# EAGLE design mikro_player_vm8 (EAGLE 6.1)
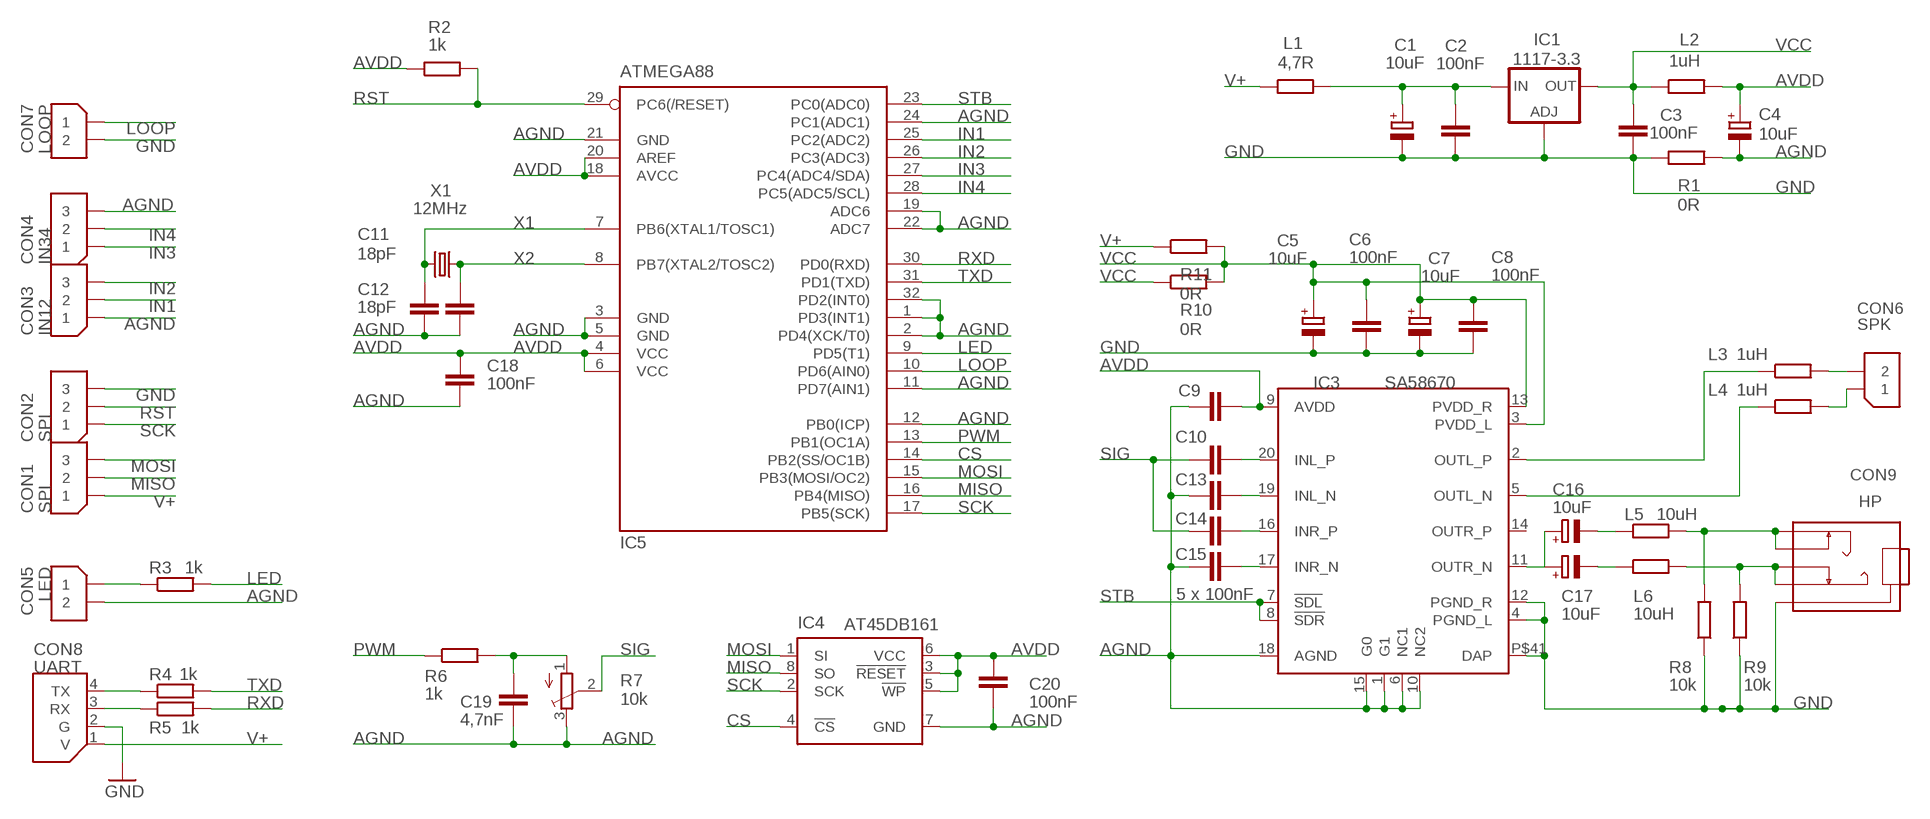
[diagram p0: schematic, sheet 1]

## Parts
C1  10uF  CPOL-EUSMCA  [SMC_A]
C2  100nF  C-EUC0805K  [C0805K]
C3  100nF  C-EUC0805K  [C0805K]
C4  10uF  CPOL-EUSMCA  [SMC_A]
C5  10uF  CPOL-EUSMCA  [SMC_A]
C6  100nF  C-EUC0805K  [C0805K]
C7  10uF  CPOL-EUSMCA  [SMC_A]
C8  100nF  C-EUC0805K  [C0805K]
C9  100nF  C-EUC0805K  [C0805K]
C10  100nF  C-EUC0805K  [C0805K]
C11  18pF  C-EUC0805K  [C0805K]
C12  18pF  C-EUC0805K  [C0805K]
C13  100nF  C-EUC0805K  [C0805K]
C14  100nF  C-EUC0805K  [C0805K]
C15  100nF  C-EUC0805K  [C0805K]
C16  10uF  CPOL-EUSMCA  [SMC_A]
C17  10uF  CPOL-EUSMCA  [SMC_A]
C18  100nF  C-EUC0805K  [C0805K]
C19  4,7nF  C-EUC0805K  [C0805K]
C20  100nF  C-EUC0805K  [C0805K]
CON1  SPI  GOLDPIN_1X3  [GOLDPIN_1X3]
CON2  SPI  GOLDPIN_1X3  [GOLDPIN_1X3]
CON3  IN12  GOLDPIN_1X3  [GOLDPIN_1X3]
CON4  IN34  GOLDPIN_1X3  [GOLDPIN_1X3]
CON5  LED  GOLDPIN_1X2  [GOLDPIN_1X2]
CON6  SPK  GOLDPIN_1X2  [GOLDPIN_1X2]
CON7  LOOP  GOLDPIN_1X2  [GOLDPIN_1X2]
CON8  UART  MOD09  [MOD09]
CON9  HP  JACK_3_5  [JACK_3_5]
IC1  1117-3.3  LD117ADT33TR  [DPACK]
IC3  SA58670  [MLF20]
IC4  AT45DB161  AT45DBXXX  [SOIC8]
IC5  ATMEGA88  MEGA8-AI  [TQFP32-08]
L1  4,7R  R-EU_R0805  [R0805]
L2  1uH  R-EU_R0805  [R0805]
L3  1uH  R-EU_R0805  [R0805]
L4  1uH  R-EU_R0805  [R0805]
L5  10uH  R-EU_R0805  [R0805]
L6  10uH  R-EU_R0805  [R0805]
R1  0R  R-EU_R0805  [R0805]
R2  1k  R-EU_R0805  [R0805]
R3  1k  R-EU_R0805  [R0805]
R4  1k  R-EU_R0805  [R0805]
R5  1k  R-EU_R0805  [R0805]
R6  1k  R-EU_R0805  [R0805]
R7  10k  TRIM_EU-SM-42/43A  [SM-42/43A]
R8  10k  R-EU_R0805  [R0805]
R9  10k  R-EU_R0805  [R0805]
R10  0R  R-EU_R0805  [R0805]
R11  0R  R-EU_R0805  [R0805]
X1  12MHz  CRYSTALHC49UP  [HC49UP]

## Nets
AGND: C4.- C9.2 C11.1 C12.1 C13.1 C15.1 C18.2 C19.2 C20.1 CON3.P$1 CON4.P$3 CON5.2 IC3.1(G1) IC3.6(NC1) IC3.10(NC2) IC3.15(G0) IC3.18(AGND) IC4.7(GND) IC5.1(PD3(INT1)) IC5.2(PD4(XCK/T0)) IC5.3(GND) IC5.5(GND) IC5.11(PD7(AIN1)) IC5.12(PB0(ICP)) IC5.19(ADC6) IC5.21(GND) IC5.22(ADC7) IC5.24(PC1(ADC1)) IC5.32(PD2(INT0)) R1.2 R7.3(E)
AVDD: C4.+ C9.1 C18.1 C20.2 IC3.9(AVDD) IC4.3(!RESET) IC4.5(!WP) IC4.6(VCC) IC5.4(VCC) IC5.6(VCC) IC5.18(AVCC) IC5.20(AREF) L2.2 R2.1
CS: IC4.4(!CS) IC5.14(PB2(SS/OC1B))
GND: C1.- C2.2 C3.2 C5.- C6.2 C7.- C8.2 CON2.P$3 CON7.2 CON8.2(G) CON9.G IC1.1(ADJ) IC3.4(PGND_L) IC3.12(PGND_R) IC3.P$41(DAP) R1.1 R8.1 R9.1
IN1: CON3.P$2 IC5.25(PC2(ADC2))
IN2: CON3.P$3 IC5.26(PC3(ADC3))
IN3: CON4.P$1 IC5.27(PC4(ADC4/SDA))
IN4: CON4.P$2 IC5.28(PC5(ADC5/SCL))
LED: IC5.9(PD5(T1)) R3.2
LOOP: CON7.1 IC5.10(PD6(AIN0))
MISO: CON1.P$2 IC4.8(SO) IC5.16(PB4(MISO))
MOSI: CON1.P$3 IC4.1(SI) IC5.15(PB3(MOSI/OC2))
N$1: CON8.4(TX) R4.1
N$2: CON8.3(RX) R5.1
N$5: C10.2 IC3.20(INL_P)
N$6: CON5.1 R3.1
N$7: C13.2 IC3.19(INL_N)
N$8: C14.2 IC3.16(INR_P)
N$9: C15.2 IC3.17(INR_N)
N$12: C17.- L6.1
N$13: C16.- L5.1
N$14: CON6.2 L3.2
N$15: CON6.1 L4.2
N$16: CON9.R CON9.RW L5.2 R8.2
N$17: IC3.2(OUTL_P) L3.1
N$18: IC3.5(OUTL_N) L4.1
N$19: C19.1 R6.2 R7.1(A)
N$22: CON9.L CON9.LW L6.2 R9.2
N$32: C16.+ C17.+ IC3.11(OUTR_N)
PVCC: C1.+ C2.1 IC1.3(IN) L1.2
PWM: IC5.13(PB1(OC1A)) R6.1
RST: CON2.P$2 IC5.29(PC6(/RESET)) R2.2
RXD: IC5.30(PD0(RXD)) R5.2
SCK: CON2.P$1 IC4.2(SCK) IC5.17(PB5(SCK))
SIG: C10.1 C14.1 R7.2(S)
STB: IC3.7(!SDL) IC3.8(!SDR) IC5.23(PC0(ADC0))
TXD: IC5.31(PD1(TXD)) R4.2
V+: CON1.P$1 CON8.1(V) L1.1 R11.1
VCC: C3.1 C5.+ C6.1 C7.+ C8.1 IC1.4(OUT) IC3.3(PVDD_L) IC3.13(PVDD_R) L2.1 R10.1 R10.2 R11.2
X1: C11.2 IC5.7(PB6(XTAL1/TOSC1)) X1.2
X2: C12.2 IC5.8(PB7(XTAL2/TOSC2)) X1.1
Unconnected: IC3.14(OUTR_P)

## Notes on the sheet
- 5 x 100nF

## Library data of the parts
C1 C4 C5 C7 C16 C17 = rcl:CPOL-EU: POLARIZED CAPACITOR, European symbol
C2 C3 C6 C8-C15 C18-C20 = rcl:C-EU: CAPACITOR, European symbol
CON1-CON4 = DS:GOLDPIN_1X3
CON5-CON7 = DS:GOLDPIN_1X2
CON8 = DS:MOD09
CON9 = Jacki:JACK_3_5
IC1 = v-reg:LD117A?*: Low drop fixed and adjustable positive voltage regulators 1 A Source: http://www.st.com/stonline/products/literature/ds/7194/ld1117axx.pdf
IC3 = DS:SA58670
IC4 = DS:AT45DBXXX
IC5 = atmel:MEGA8: MICROCONTROLLER 8 Kbytes FLASH, 1 kbytes SRAM, 512 bytes EEPROM, USART, 6-channel 10 bit ADC, 2-channel 8 bit ADC Pin compatible with Atmega48, ATMega88, ATMega168 Source: avr.lbr; MPN: ATMEGA8-16AU; OC_FARNELL: 9171371; OC_NEWARK: 73M8863
L1-L6 R1-R6 R8-R11 = rcl:R-EU_: RESISTOR, European symbol
R7 = pot:TRIM_EU-: POTENTIOMETER
X1 = crystal:CRYSTAL: CRYSTAL; OC_FARNELL: unknown; OC_NEWARK: unknown

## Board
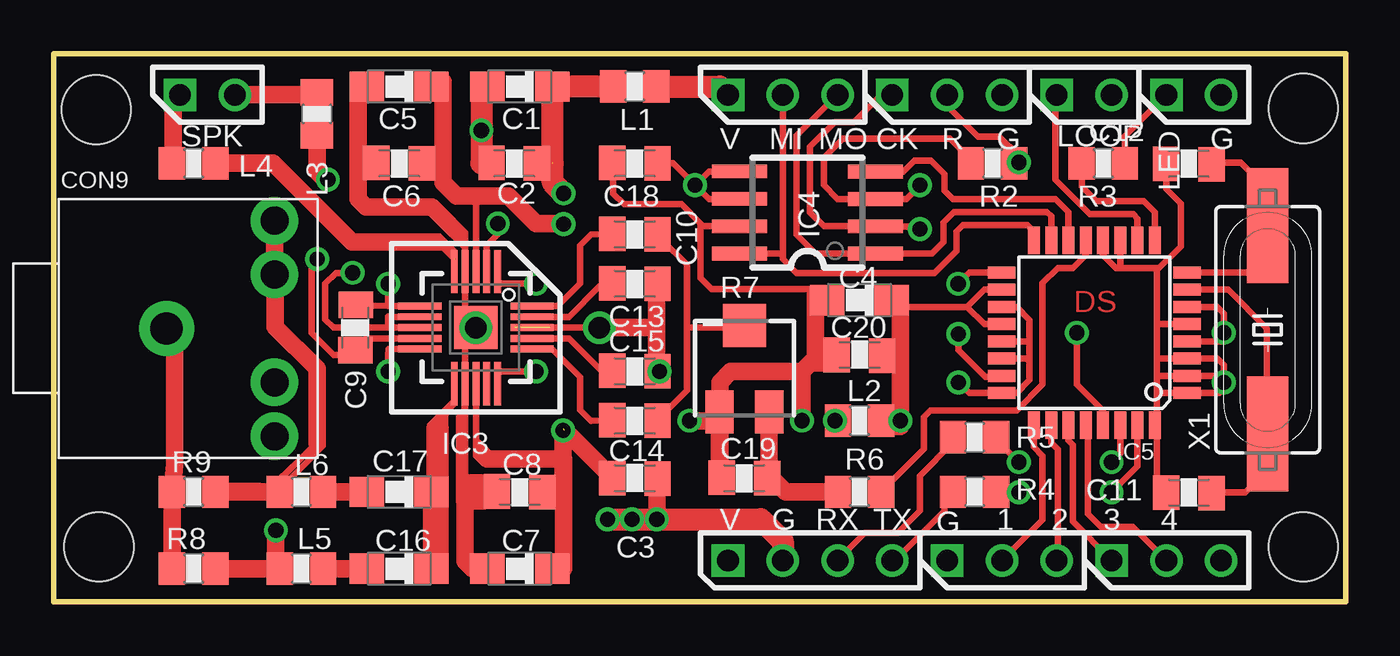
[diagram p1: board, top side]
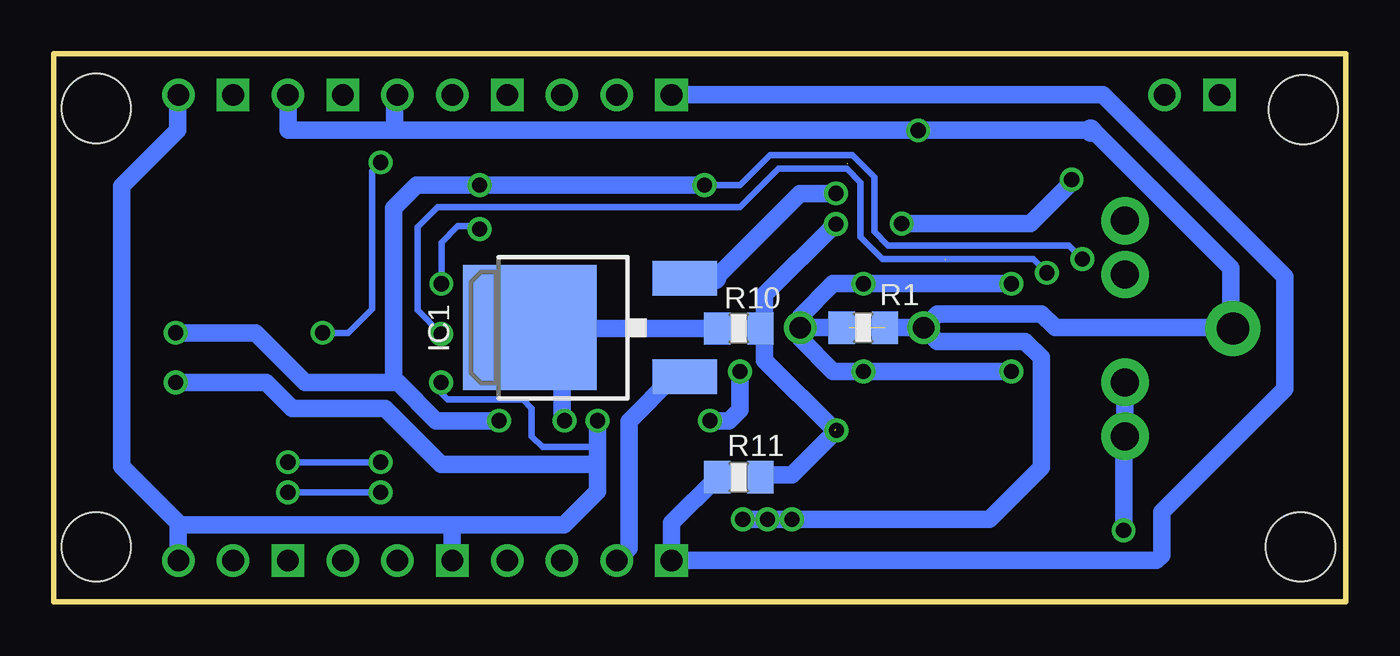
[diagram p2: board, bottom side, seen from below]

Size 59.87 x 25.42 mm. Coordinates in mm from the lower left corner, seen from the top.
Outline: 0,0 59.87,0 59.87,25.42 0,25.42 0,0
Copper layers (1*16): Top 0.035mm / dielectric 1.5mm / Bottom 0.035mm
Design rules: minimum track width 10mil, minimum drill 24mil, track to track 8mil, track to pad 8mil, pad to pad 8mil, via to via 8mil, smd to smd 8mil, copper to edge 40mil, drill to drill 8mil, minimum pad ring 10mil, minimum via ring 8mil, stop-mask expansion 4mil, vias tented up to drill 0mil, thermal gap 10mil
Holes 3.2 mm at 57.91,2.57 1.96,22.83 2.08,2.57 57.91,22.89

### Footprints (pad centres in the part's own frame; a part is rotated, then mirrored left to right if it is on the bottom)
SMC_A = smd 1.6 x 1.4: + -1.5,0; - 1.5,0
C0805K = smd 1.219 x 1.6: 1 -1.051,0; 2 1.051,-0.025
GOLDPIN_1X3 = drill 1 square: P$1 -2.54,0 | drill 1: P$2 0,0; P$3 2.54,0
GOLDPIN_1X2 = drill 1 square: 1 -1.27,0 | drill 1: 2 1.27,0
MOD09 = drill 1 square: 1 0,-5.08 | drill 1: 2 0,-2.54; 3 0,0; 4 0,2.54
JACK_3_5 = drill 1.5 pad 2.54: G -1.4,0 | drill 1.3 pad 2.2: L 3.6,5; LW 3.6,2.5; R 3.6,-5; RW 3.6,-2.5
DPACK = smd 1.6 x 3: 1 -2.28,-4.8; 3 2.28,-4.8 | smd 5.8 x 6.2: 4 0,2.38
MLF20 = smd 0.32 x 2: 1 -1,-2.6; 2 -0.5,-2.6; 3 0,-2.6; 4 0.5,-2.6; 5 1,-2.6; 11 1,2.6; 12 0.5,2.6; 13 0,2.6; 14 -0.5,2.6; 15 -1,2.6 | smd 2 x 0.32: 6 2.6,-1; 7 2.6,-0.5; 8 2.6,0; 9 2.6,0.5; 10 2.6,1; 16 -2.6,1; 17 -2.6,0.5; 18 -2.6,0; 19 -2.6,-0.5; 20 -2.6,-1 | smd 2 x 2: P$41 0,0
SOIC8 = smd 0.635 x 2.54: 1 -1.905,-3.154; 2 -0.645,-3.154; 3 0.625,-3.154; 4 1.895,-3.154; 5 1.905,3.154; 6 0.635,3.154; 7 -0.635,3.154; 8 -1.905,3.154
TQFP32-08 = smd 1.27 x 0.559: 1 -4.293,2.8; 2 -4.293,2; 3 -4.293,1.2; 4 -4.293,0.4; 5 -4.293,-0.4; 6 -4.293,-1.2; 7 -4.293,-2; 8 -4.293,-2.8; 17 4.293,-2.8; 18 4.293,-2; 19 4.293,-1.2; 20 4.293,-0.4; 21 4.293,0.4; 22 4.293,1.2; 23 4.293,2; 24 4.293,2.8 | smd 0.559 x 1.27: 9 -2.8,-4.293; 10 -2,-4.293; 11 -1.2,-4.293; 12 -0.4,-4.293; 13 0.4,-4.293; 14 1.2,-4.293; 15 2,-4.293; 16 2.8,-4.293; 25 2.8,4.293; 26 2,4.293; 27 1.2,4.293; 28 0.4,4.293; 29 -0.4,4.293; 30 -1.2,4.293; 31 -2,4.293; 32 -2.8,4.293
R0805 = smd 1.219 x 1.5: 1 -1.001,0; 2 1.001,0
SM-42/43A = smd 2 x 1.3: 1 2,1.15; 3 2,-1.15 | smd 2 x 2: 2 -2,0
HC49UP = smd 5.334 x 1.93: 1 -4.826,0; 2 4.826,0

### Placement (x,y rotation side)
C1  21.59,23.9 180 top
C2  21.34,20.35 180 top
C3  26.92,5.74 0 top
C4  37.34,14 180 top
C5  16,23.9 180 top
C6  16,20.35 180 top
C7  21.59,1.55 180 top
C8  21.59,5.11 180 top
C9  13.97,12.73 90 top
C10  26.92,17.04 180 top
C11  52.6,5.07 0 top
C12  52.6,20.33 0 top
C13  26.92,14.76 180 top
C14  26.92,8.41 180 top
C15  26.92,10.69 180 top
C16  16,1.55 180 top
C17  16,5.11 180 top
C18  26.92,20.35 180 top
C19  32,5.74 180 top
C20  37.34,11.46 0 top
CON1  33.78,23.52 0 top
CON2  41.4,23.52 0 top
CON3  43.94,1.93 0 top
CON4  51.56,1.93 0 top
CON5  52.83,23.52 0 top
CON6  7.11,23.52 0 top
CON7  47.75,23.52 0 top
CON8  36.32,1.93 270 top
CON9  6.62,12.69 0 top
IC1  35.43,12.73 90 bottom
IC3  19.56,12.73 180 top
IC4  34.93,18.06 90 top
IC5  48.22,12.49 180 top
L1  26.92,23.9 180 top
L2  37.34,8.41 0 top
L3  12.19,22.63 90 top
L4  6.48,20.35 180 top
L5  11.48,1.55 180 top
L6  11.48,5.11 180 top
R1  22.35,12.73 180 bottom
R2  43.51,20.35 0 top
R3  48.64,20.35 180 top
R4  42.67,5.11 0 top
R5  42.67,7.65 0 top
R6  37.34,5.11 180 top
R7  32,10.82 270 top
R8  6.48,1.55 0 top
R9  6.48,5.11 0 top
R10  28.12,12.69 180 bottom
R11  28.12,5.79 0 bottom
X1  56.26,12.63 270 top

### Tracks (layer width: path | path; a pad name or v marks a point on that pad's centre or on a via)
AGND  (via drill 0.7, 1)
  Top 0.305: IC3.10 15.51,11.73 15.49,11.46 v15.49,10.69 | IC3.6 15.51,13.73 15.49,13.74 | 15.49,13.74 v15.49,14.76 | C9.2 15.48,13.73 15.49,13.74 | IC3.15 20.56,10.68 20.57,10.69 v22.35,10.69 | IC3.1 20.56,14.77 20.57,14.76 v22.35,14.76 | IC3.18 v25.27,12.73 | IC4.7 29.97,17.42 | 29.97,17.42 29.97,15.01 30.48,14.5 35.31,14.5 35.31,14.25 | 29.97,17.42 29.97,17.55 29.08,18.44 26.42,18.44 25.91,18.95 25.91,20.33 C18.2 | C12.1 51.55,19.16 52.22,18.49 52.22,16.49 51.22,15.49 51.12,15.49 | 51.12,15.49 51.12,12.89 | 51.52,5.1 C11.1 51.12,5.5 51.12,8.29 | IC5.5 51.12,12.89 | IC5.21 45.22,12.09 | 45.22,12.09 45.22,11.19 | 45.22,11.19 45.22,10.29 44.62,9.69 IC5.24 42.42,9.69 v41.92,10.19 | IC5.12 48.62,16.09 49.22,15.49 49.42,15.49 | 49.42,15.49 51.12,15.49 | IC5.11 49.42,15.49 | 45.22,12.09 45.22,13.09 44.62,13.69 IC5.19 | IC5.22 45.12,11.29 45.22,11.19 | 51.12,12.89 51.12,11.29 | 51.12,11.29 51.12,10.49 | 51.12,10.49 51.12,9.69 | 51.12,9.69 51.12,8.29 | IC5.32 51.12,8.29 | 54.22,10.39 v54.22,10.19 54.22,9.89 54.02,9.69 IC5.1 51.12,9.69 | 54.22,10.39 54.22,10.99 53.92,11.29 IC5.3 51.12,11.29 | 54.22,10.39 54.12,10.49 IC5.2 51.12,10.49
  Top 0.813: 27.94,14.76 C13.1 | 27.94,10.69 C15.1 v28.07,10.69 27.94,10.82 27.94,12.73 | 27.92,14.74 27.94,14.76 | 30.85,6.62 R7.3 30.86,8.7 30.86,10.19 31.37,10.69 34.67,10.69 | C19.2 30.85,5.89 30.85,6.62 | v29.46,8.41 30.86,8.41 30.86,6.63 30.85,6.62 | C4.- 35.84,14.25 35.31,14.25 35.31,11.07 36.32,11.07 36.34,11.09 C20.1 35.43,11.46 34.67,10.69 | 34.67,10.69 v34.67,8.41 | v25.27,12.73 27.94,12.73 | 27.94,12.73 27.94,14.76
  Bottom 0.305: v41.92,10.19 41.92,9.69 41.62,9.39 38.12,9.39 37.72,8.99 37.72,7.69 37.22,7.19 34.87,7.19 34.67,7.39
  Bottom 0.813: v15.49,14.76 v22.35,14.76 23.75,14.76 25.27,13.23 v25.27,12.73 | v15.49,10.69 v22.35,10.69 23.75,10.69 25.27,12.22 v25.27,12.73 | R1.2 v25.27,12.73 | v28.07,10.69 28.07,8.92 28.58,8.41 v29.46,8.41 | v34.67,8.41 34.67,7.39 34.67,6.49 | 34.67,6.49 34.67,5.14 36.22,3.59 41.32,3.59 | 41.32,3.59 54.05,3.59 | CON3.P$1 41.4,3.47 41.32,3.59 | 54.05,3.59 54.05,3.61 56.72,6.29 56.72,19.29 54.12,21.89 54.12,23.5 CON5.2 | CON4.P$3 54.1,3.53 54.05,3.59 | v54.22,10.19 50.02,10.19 48.82,8.99 44.52,8.99 41.92,6.39 34.77,6.39 34.67,6.49
AVDD  (via drill 0.7)
  Top 0.305: C9.1 14.47,12.23 IC3.9 14.74,12.23 13.97,11.46 12.95,11.46 11.94,12.47 11.94,15.65 v12.19,15.9 | v29.72,19.33 30.35,18.69 IC4.6 | v40.13,19.33 39.52,18.68 IC4.3 38.07,18.69 36.32,18.69 35.69,19.33 35.69,20.6 36.58,21.49 41.53,21.49 42.48,20.53 R2.1 | IC4.5 30.35,19.96 v29.72,19.33 | C18.1 28.7,20.35 v29.72,19.33 | IC5.6 53.92,13.69 54.22,13.39 v54.22,12.49 54.22,12.09 IC5.4 | IC5.18 43.12,14.49 42.32,13.69 | 42.32,13.69 39.24,13.69 | IC5.20 43.12,12.89 42.32,13.69
  Top 0.813: C20.2 38.34,11.09 38.48,11.07 39.24,11.07 | 39.24,11.07 39.24,13.69 39.24,13.97 C4.+ 39.24,14 | 38.35,8.15 38.29,8.22 L2.2 38.54,8.15 39.24,8.15 v39.24,8.41 39.24,11.07
  Bottom 0.305: v12.19,15.9 12.83,16.54 21.21,16.54 21.84,17.17 21.84,19.71 22.86,20.73 26.67,20.73 28.07,19.33 v29.72,19.33
  Bottom 0.813: v29.72,19.33 v40.13,19.33 43.05,19.33 44.12,18.26 44.12,10.19 | v39.24,8.41 42.14,8.41 43.92,10.19 44.12,10.19 | 44.12,10.19 48.22,10.19 50.52,12.49 v54.22,12.49
CS
  Top 0.305: IC4.4 39.37,19.96 39.88,20.47 40.64,20.47 41.27,19.84 41.27,19.08 41.67,18.69 46.42,18.69 47.02,18.09 IC5.14
GND  (via drill 0.7, 1)  (1 unrouted)
  Top 0.305: 18.8,4.86 19.06,4.6 | 19.06,5.11 18.8,5.37 18.8,8.56 19.06,8.82 IC3.12 19.06,12.23 IC3.P$41 | IC3.P$41 19.56,12.47 19.05,11.96 | IC3.P$41 19.06,13.23 IC3.4 19.06,17.14 18.29,17.91 18.29,17.81 18.16,17.68
  Top 0.813: C7.- 19.41,1.55 19.06,1.9 19.06,4.6 19.06,5.11 C8.2 | R8.1 R9.1 5.59,6.38 5.59,12.32 CON9.G | 14.1,20.35 14.1,18.69 14.48,18.31 17.53,18.31 18.16,17.68 18.29,17.55 | 14.1,20.35 14.1,23.88 C5.- | C6.2 14.1,20.35 | C3.2 27.92,3.85 v27.94,3.84
  Top 1.016: v25.65,3.84 v26.8,3.84 v27.94,3.84 32.77,3.84 33.78,2.82 CON8.2 | C1.- 19.94,23.9 19.81,24.03 v19.81,21.87 19.81,20.36 | 19.81,20.36 C2.2 19.81,20.35 19.81,20.36
  Bottom 0.813: IC3.P$41 18.92,12.09 14.86,12.09 14.1,11.33 14.1,6.25 16.51,3.84 v25.65,3.84 v27.94,3.84 | IC3.P$41 18.92,13.36 14.1,13.36 13.46,12.73 5.26,12.73 | 11.81,21.87 v19.81,21.87 44.17,21.87 44.07,22 | 44.07,22 44.07,23.39 CON2.P$3 | CON7.2 49.02,21.87 44.2,21.87 44.07,22 | 11.8,21.86 11.69,21.86 5.32,15.49 5.32,12.79 | 22.99,12.73 IC3.P$41 | IC1.1 31.16,10.45 33.22,8.39 33.22,2.49 CON8.2
  Bottom 1.016: 11.8,21.86 11.81,21.87 | 5.32,12.79 CON9.G 5.26,12.73
  other vias: 19.56,12.73
IN1
  Top 0.305: IC5.25 45.42,7.19 45.82,6.79 45.82,3.81 CON3.P$2
IN2
  Top 0.305: IC5.26 46.22,7.39 46.52,7.09 46.52,1.89 CON3.P$3
IN3
  Top 0.305: IC5.27 47.02,7.49 47.22,7.29 47.22,3.73 CON4.P$1
IN4
  Top 0.305: IC5.28 47.82,7.69 47.92,7.59 47.92,4.09 48.52,3.49 50.01,3.49 CON4.P$2
LED
  Top 0.305: IC5.9 51.02,18.09 50.52,18.59 48.32,18.59 47.64,19.27 R3.2
LOOP
  Top 0.305: IC5.10 50.22,17.79 50.02,17.99 48.02,17.99 46.42,19.59 46.42,23.46 CON7.1
MISO
  Top 0.305: CON1.P$2 33.78,16.15 | 33.78,16.15 IC4.8 | 33.78,16.15 33.78,15.9 34.42,15.27 40.8,15.27 41.82,16.29 41.82,17.19 42.12,17.49 45.12,17.49 45.41,17.19 IC5.16
MOSI
  Top 0.305: CON1.P$3 34.42,21.62 34.42,17.04 35.31,16.15 IC4.1 40.69,16.15 41.22,16.69 41.22,17.59 41.72,18.09 46.02,18.09 46.22,17.89 IC5.15
N$1
  Top 0.305: CON8.4 38.99,1.93 41.27,4.22 41.27,4.66 R4.1
N$2
  Top 0.305: CON8.3 37.59,3.2 39.12,3.2 40.13,4.22 40.13,5.86 41.67,7.39 R5.1
N$5
  Top 0.305: IC3.20 23.35,13.73 24.38,14.76 24.38,16.54 24.89,17.04 C10.2
N$6
  Top 0.305: R3.1 49.64,21.6 CON5.1
N$7
  Top 0.305: IC3.19 23.87,13.23 25.27,14.63 C13.2
N$8
  Top 0.305: IC3.16 23.1,11.73 24.38,10.44 24.38,8.92 24.89,8.41 C14.2
N$9
  Top 0.305: IC3.17 23.87,12.23 25.4,10.69 C15.2
N$10
  Top 0.305: 19.05,16.15 19.05,16.43 17.88,17.6 18.03,17.75 18.09,17.75 19,16.84
N$12
  Top 0.813: L6.1 C17.-
N$13
  Top 0.813: L5.1 C16.-
N$14
  Top 0.813: CON6.2 12.13,23.52 L3.2
N$15
  Top 0.813: CON6.1 5.53,23.21 5.53,20.4 L4.2
N$16  (via drill 0.7)
  Top 0.406: L5.2 10.16,1.55
  Top 0.813: R8.2 10.16,1.55 10.29,1.55 v10.29,3.33
  Bottom 0.813: v10.29,3.33 10.29,7.62 CON9.R CON9.RW
N$17  (via drill 0.7)
  Top 0.305: IC3.2 20.06,16.53 20.57,17.04 v20.57,17.55
  Top 0.813: L3.1 12.19,19.96 12.7,19.46 v12.7,19.58
  Bottom 0.813: v20.57,17.55 14.6,17.55 12.7,19.46 v12.7,19.58
N$18  (1 unrouted)
  Top 0.305: 17.27,16.46 17.27,16.43 18.03,16.43 18.57,15.9 18.57,15.98 | 17.37,16.69 17.4,16.69 17.4,16.94 17.88,16.94 18.57,16.26 18.57,15.98 | 18.57,15.98 17.78,16.76 | IC3.5 18.56,15.88 18.54,15.9
  Top 0.813: L4.1 10.16,20.35 13.82,16.69 17.37,16.69
N$19
  Top 0.813: 33.15,5.89 C19.1 | 33.31,8.66 R7.1 33.15,5.89 | 33.15,5.89 33.15,5.86 33.91,5.11 R6.2
N$20
  Top 0.305: 11.81,6.76 12.06,6.86 12.45,7.24 12.45,7.26
N$22
  Top 0.305: 12.19,7.36 12.06,7.26 10.67,5.87 10.57,5.34 | 10.57,5.34 10.67,5.55 L6.2 | 10.41,5.54 10.41,5.67 12.19,7.35 | 12.32,7.14 11.96,6.74 10.57,5.34
  Top 0.813: 7.87,5.11 L6.2 9.5,5.14 7.91,5.14 7.87,5.11 | 7.87,5.11 R9.2 | 12.19,7.35 12.19,7.36 12.19,10.82 10.25,12.76 10.25,15.16 CON9.LW CON9.L
N$23
  Top 0.305: 18.54,9.27 18.54,9.25
N$25
  Top 0.305: 19.05,8.99 19.05,8.86 18.8,8.61
N$26
  Top 0.305: 19.66,6.99 19.96,6.68
N$32
  Top 0.305: 17.48,8 17.42,8 17.42,8.2 18.49,9.27 18.54,9.27 18.54,9.22 18.56,9.19 | IC3.11 18.56,9.19 | 18.56,9.19 18.14,8.76 | 18.14,8.76 17.53,8.15 17.53,5.13 C17.+ | 18.14,8.76 18.14,8.1 17.78,8.1 17.98,8.31
  Top 0.813: C17.+ C16.+
PVCC  (via drill 0.7)  (1 unrouted)
  Top 0.813: 23.09,20.34 C2.1 | 22.73,20.35 22.73,20.47 22.23,20.47
  Top 1.016: L1.2 C1.+ 23.09,20.34 | 22.73,20.35 23.11,20.35 23.11,19.46 v23.62,18.95
  Bottom 0.813: 29.23,15.01 25.28,18.95 v23.62,18.95
  Bottom 1.016: IC1.3 29.23,15.01
PWM
  Top 0.305: IC5.13 47.82,16.09 47.22,15.49 46.52,15.49 45.82,14.79 45.82,10.09 44.62,8.89 40.62,8.89 40.32,8.59 40.32,7.09 R6.1
RST  (via drill 0.7)
  Top 0.305: CON2.P$2 41.42,23.5 41.42,22.99 42.82,21.59 43.82,21.59 44.67,20.74 | 44.67,20.74 44.52,20.39 v44.72,20.39 | v47.42,12.49 47.42,10.09 48.62,8.89 IC5.29 | R2.2 44.51,20.57 44.67,20.74
  Bottom 0.305: v44.72,20.39 45.12,19.99 45.12,13.59 46.22,12.49 v47.42,12.49
RXD  (via drill 0.7)
  Top 0.305: R5.2 43.67,7.53 v44.72,6.49 | IC5.30 49.42,6.89 v49.02,6.49
  Bottom 0.305: v44.72,6.49 v49.02,6.49
SCK  (via drill 0.7)
  Top 0.305: CON2.P$1 38.35,23.52 37.08,22.25 36.2,22.25 35.05,21.11 35.05,18.06 35.69,17.42 38.07,17.42 IC4.2 40.02,17.41 v40.13,17.3 | IC5.17 42.44,15.29 v41.91,14.76
  Bottom 0.305: v41.91,14.76 41.91,16.66 41.15,17.42 40.26,17.42 v40.13,17.3
SIG
  Top 0.305: C10.1 28.19,16.79 29.34,15.65 29.34,12.73 | 29.34,12.73 29.34,9.82 28.19,8.66 C14.1 | R7.2 32,12.73 29.34,12.73
STB  (via drill 0.7)
  Top 0.305: IC3.8 15.49,12.73 | IC3.7 15.5,13.23 15.49,13.23 15.49,12.73 | 15.49,12.73 12.95,12.73 12.57,13.11 12.57,14.76 13.08,15.27 v13.84,15.27 | IC5.23 43.88,10.43 43.17,10.43 41.92,11.69 v41.92,12.43
  Bottom 0.305: v13.84,15.27 14.48,15.9 21.46,15.9 22.48,16.92 22.48,19.46 23.11,20.09 26.29,20.09 28.07,18.31 42.09,18.31 43.02,17.39 43.02,13.53 v41.92,12.43
TXD  (via drill 0.7)
  Top 0.305: R4.2 44.2,5.11 44.22,5.09 v44.72,5.09 | v49.02,5.09 50.22,6.29 IC5.31
  Bottom 0.305: v44.72,5.09 v49.02,5.09
V+
  Top 1.016: L1.1 30.86,23.9 CON1.P$1
  Bottom 0.813: CON1.P$1 11.26,23.52 2.82,15.09 2.82,9.89 8.52,4.19 8.52,2.17 8.76,1.93 CON8.1 31.24,3.67 R11.1
VCC  (via drill 0.7)  (1 unrouted)
  Top 0.305: IC3.13 19.56,7.52 | 19.56,7.52 20.45,6.63 | 19.56,7.52 19.56,6.78 19.91,6.43 20.02,6.43 20.07,6.48 20.07,6.63 | IC3.3 19.56,18.82
  Top 0.813: 23.62,5.11 23.62,1.55 C7.+ | C8.1 23.62,5.11 | 18.03,19.51 18.03,20.35 | 18.03,20.35 18.03,24.13 C5.+ | C6.1 18.03,20.35 | 23.62,5.11 23.62,5.87 | 23.62,5.87 23.62,6.63 20.07,6.63 19.81,6.88 | 18.03,19.51 18.06,19.46 | v23.62,17.53 23.62,17.55 22.35,17.55 21.08,18.82 19.56,18.82 18.67,18.82 18.03,19.46 18.03,19.51 | v23.6,7.95 23.6,5.89 23.62,5.87 | C3.1 25.91,5.74 23.62,8.03 | L2.1 v36.2,8.41
  Bottom 0.813: v23.62,17.53 23.62,17.55 26.92,14.25 26.92,12.49 | v36.2,8.41 36.32,8.53 36.32,12.76 37.23,12.74 IC1.4 | 26.92,12.49 26.92,11.2 23.67,7.95 v23.6,7.95 25.66,5.89 26.92,5.89 27.02,5.79 R11.2 | 26.92,12.49 R10.1 R10.2 37.18,12.69
  Bottom 1.016: 37.18,12.69 37.23,12.74
X1
  Top 0.305: IC5.7 54.42,14.49 56.22,12.69 56.22,6.79 | 56.22,6.79 56.22,6.09 55.22,5.09 53.7,5.09 C11.2 | X1.2 56.26,6.82 56.22,6.79
X2
  Top 0.305: IC5.8 56.12,15.29 56.22,15.39 56.22,18.79 | 56.22,18.79 56.22,19.19 55.02,20.39 53.67,20.39 C12.2 | X1.1 56.26,18.75 56.22,18.79
(copper drawn outside any net)
  shapes: Top area x6

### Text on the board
Top: DS
tPlace: SPK | LOOP | LED | V | MI | MO | CK | R | G | G | V | G | RX | TX | G | 1 | 2 | 3 | 4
